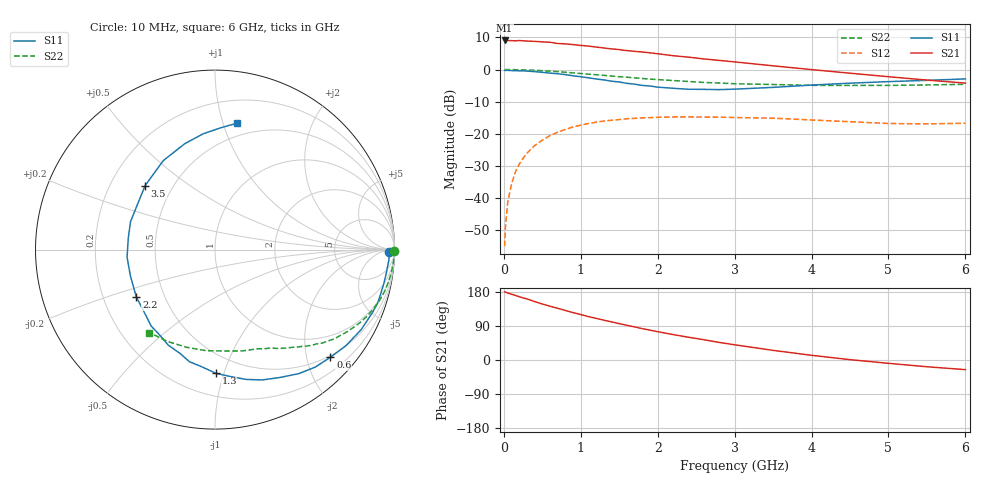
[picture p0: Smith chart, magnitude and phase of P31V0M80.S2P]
! SIEMENS Small Signal Semiconductors
! BFP181
! Si NPN RF Bipolar Junction Transistor in SOT143
! VCE = 1 V  IC = 0.8 mA
! Common Emitter S-Parameters:  March  1996
# GHz  S  MA  R  50
!  f  S11  S21  S12  S22
! GHz  MAG  ANG  MAG  ANG  MAG  ANG  MAG  ANG
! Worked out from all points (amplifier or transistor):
!   36 points, 10 MHz to 6 GHz, reference 50 ohm
!   highest |S21| = 9.0 dB at 10 MHz (marker M1)
!   |S21| within 3 dB of that: start of sweep to 1.55 GHz
!   unconditionally stable (mu >= 1): 3.165 GHz to end of sweep
!   at 250 MHz: K = 0.09, MSG = 18.3 dB, |S12| = -27.6 dB
!   at 1.4 GHz: K = 0.49, MSG = 11.1 dB, |S12| = -15.8 dB
!   at 6 GHz: K = 1.41, MAG = 2.4 dB, |S12| = -16.7 dB
!   S11 on the Smith chart (normalised r, x): 10 MHz: 51, -21; 600 MHz: 0.46, -2.46; 1.3 GHz: 0.36, -0.94; 2.2 GHz: 0.35, -0.25; 3.5 GHz: 0.35, +0.35; 6 GHz: 0.39, +1.12
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0.01  0.9668 -0.8  2.83 179.7  0.0018 89.2  0.9993 -0.3
0.02  0.971 -1.4  2.815 179.4  0.0035 77.6  0.998 -0.8
0.05  0.9706 -3.4  2.821 176.8  0.0086 92.1  0.9979 -1.8
0.1  0.9638 -7.5  2.807 173.7  0.0166 83.8  0.9975 -3.5
0.15  0.9599 -11.1  2.793 170.4  0.0255 81.7  0.994 -5.3
0.2  0.9555 -14.8  2.817 167.1  0.0338 80.6  0.9914 -7.1
0.3  0.945 -21.7  2.768 161.3  0.05 75.0  0.9829 -10.6
0.4  0.9287 -28.6  2.74 154.2  0.0656 70.6  0.9725 -14.0
0.6  0.8795 -43.0  2.651 142.0  0.094 61.1  0.943 -20.5
0.9  0.7994 -63.0  2.44 125.1  0.1281 48.5  0.8867 -29.1
1.1  0.7439 -76.5  2.316 114.5  0.145 40.8  0.8478 -34.2
1.3  0.6893 -89.6  2.163 105.1  0.1583 34.0  0.811 -38.8
1.5  0.6404 -102.9  2.042 95.9  0.167 28.3  0.7727 -42.8
1.8  0.5663 -123.2  1.871 82.7  0.1773 20.8  0.7265 -47.9
2.2  0.5114 -149.0  1.64 67.1  0.1833 11.9  0.6742 -54.5
2.4  0.4939 -162.5  1.558 60.1  0.1838 7.8  0.6521 -57.7
2.8  0.4873 172.7  1.386 46.4  0.1819 1.7  0.617 -63.6
3.5  0.5281 137.5  1.142 25.4  0.1754 -6.7  0.5852 -74.7
4  0.5734 120.2  0.998 12.4  0.1645 -10.5  0.5678 -84.4
4.5  0.6138 105.9  0.877 0.9  0.1546 -13.2  0.5655 -95.0
5.5  0.6789 87.4  0.686 -17.8  0.1431 -10.3  0.5758 -117.1
6  0.7156 80.0  0.615 -25.4  0.1462 -8.4  0.5895 -128.4
